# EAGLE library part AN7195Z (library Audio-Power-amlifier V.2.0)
The AN7195Z is an audio power IC developed for the sound output of car audio (dual 15 W). It is incorporating various protection circuits to protect the IC from destruction by GND-open short-circuit to GND and power supply surge which are the most important subjects of power IC protection, and the IC will largely contribute to a high reliability design of equipment.
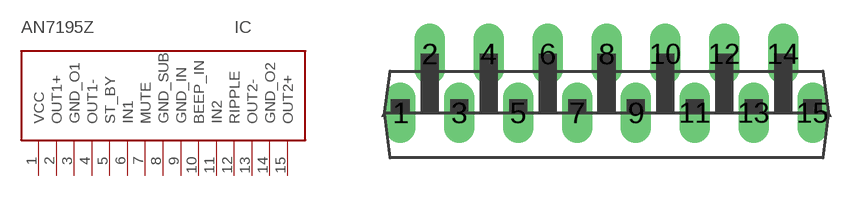
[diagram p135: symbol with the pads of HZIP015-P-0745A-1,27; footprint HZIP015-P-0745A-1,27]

Designator prefix IC

## AN7195Z  [HZIP015-P-0745A-1,27]
1  VCC  pwr
2  OUT1+  out
3  GND_O1  pwr
4  OUT1-  out
5  ST_BY  in
6  IN1  in
7  MUTE  in
8  GND_SUB  pwr
9  GND_IN  pwr
10  BEEP_IN  in
11  IN2  in
12  RIPPLE
13  OUT2-  out
14  GND_O2  pwr
15  OUT2+  out

## Footprint HZIP015-P-0745A-1,27 (pad centres in mm)
drill 0.8 long: 1 -8.89,-1.27; 2 -7.62,1.27; 3 -6.35,-1.27; 4 -5.08,1.27; 5 -3.81,-1.27; 6 -2.54,1.27; 7 -1.27,-1.27; 8 0,1.27; 9 1.27,-1.27; 10 2.54,1.27; 11 3.81,-1.27; 12 5.08,1.27; 13 6.35,-1.27; 14 7.62,1.27; 15 8.89,-1.27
